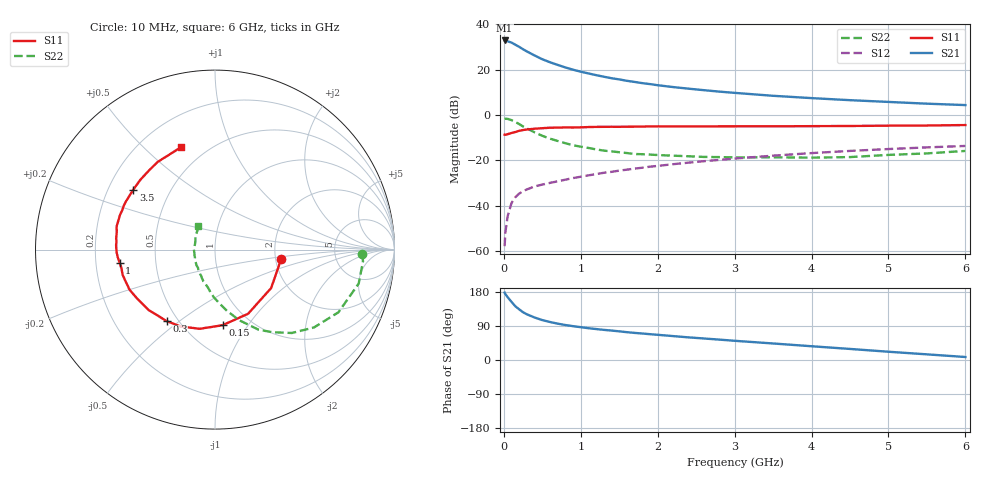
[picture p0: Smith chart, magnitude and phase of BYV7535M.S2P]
! SIEMENS Small Signal Semiconductors
! BFY420
! Si NPN RF SIEGET Grounded Emitter Transistor in MICRO-X
! VCE = 0.75 V  IC = 35 mA
! Common Emitter S-Parameters:  October  1996
# GHz  S  MA  R  50
!  f  S11  S21  S12  S22
! GHz  MAG  ANG  MAG  ANG  MAG  ANG  MAG  ANG
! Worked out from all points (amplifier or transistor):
!   36 points, 10 MHz to 6 GHz, reference 50 ohm
!   highest |S21| = 32.8 dB at 10 MHz (marker M1)
!   |S21| within 3 dB of that: start of sweep to 208.7 MHz
!   unconditionally stable (mu >= 1): start of sweep to 25.36 MHz; 979.9 MHz to end of sweep
!   at 250 MHz: K = 0.49, MSG = 31.2 dB, |S12| = -33.5 dB
!   at 1.4 GHz: K = 1.10, MAG = 18.7 dB, |S12| = -25.0 dB
!   at 6 GHz: K = 1.16, MAG = 6.6 dB, |S12| = -13.6 dB
!   S11 on the Smith chart (normalised r, x): 10 MHz: 2.13, -0.27; 150 MHz: 0.75, -0.77; 300 MHz: 0.43, -0.45; 1 GHz: 0.30, -0.06; 3.5 GHz: 0.31, +0.30; 6 GHz: 0.37, +0.66
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0.01  0.3703 -8.4  43.78 177.8  0.0013 102.6  0.8215 -1.6
0.02  0.3668 -14.8  43.42 173.8  0.0026 90.0  0.8272 -4.5
0.05  0.3792 -34.4  41.91 165.6  0.006 80.6  0.8226 -13.3
0.1  0.4022 -62.7  39.3 153.3  0.0116 70.2  0.7715 -26.9
0.15  0.4234 -84.3  35.21 141.7  0.0156 63.2  0.7016 -38.2
0.2  0.4494 -100.9  31.66 133.6  0.0187 60.5  0.6322 -47.3
0.25  0.469 -114.1  28.02 126.0  0.0211 57.0  0.5605 -55.2
0.3  0.4807 -124.0  25.07 120.5  0.0231 55.2  0.5077 -61.5
0.4  0.5001 -137.7  20.44 112.1  0.0268 53.1  0.4155 -71.1
0.5  0.5129 -148.1  16.9 105.3  0.0295 52.6  0.349 -78.8
0.6  0.5258 -154.8  14.49 100.3  0.0321 52.8  0.3022 -85.0
0.7  0.5286 -160.2  12.68 95.9  0.0348 54.1  0.2687 -90.9
0.8  0.5335 -164.8  11.14 92.3  0.0378 53.9  0.2398 -95.9
1  0.5361 -172.2  8.999 86.6  0.0439 55.0  0.2013 -104.7
1.1  0.5438 -175.6  8.228 83.9  0.047 55.8  0.1886 -110.0
1.3  0.5501 179.4  6.965 79.5  0.0536 56.0  0.1647 -117.9
1.6  0.5543 173.4  5.668 73.4  0.0628 55.6  0.1457 -129.5
2.2  0.5622 163.1  4.127 63.1  0.0828 53.3  0.1275 -148.1
3.5  0.5645 143.8  2.651 43.6  0.1275 44.3  0.1175 180.0
4.5  0.5739 130.1  2.123 29.2  0.1623 34.5  0.1188 157.0
5.5  0.588 115.0  1.778 14.9  0.1941 23.8  0.1431 133.5
6  0.602 108.1  1.656 7.9  0.2088 18.5  0.1621 124.6
